| IBIS file generated by GenIBIS323.exe Version 3.23
|   TDA2Ex_23mm_abc
[IBIS ver]   5.0
[File name]   TDA2Ex_23mm_abc.ibs
[File Rev]   1.0.0
[Date]   Mon Apr 21, 2014, 15:13:32
[Source]   Data created at Texas Instruments
[Notes]   TDA2Ex_23mm 23mm IBIS Model Revision History
   Version 1.0.0, April 21, 2014
   - Initial Release
   Note 1) Checked by IBISCHK5.
   Note 2) Interfaces Included in this TDA2Ex_23mm 23x23 IBIS Model
   - EMIF1
   - GPIO6
   - GPMC
   - CSI
   - VIP2
   - DSS
   - HDMI1
   - RGMII
   - USB1,2
   - XREFCLK
   - McASP1,2,3,4,5
   - MMC1,3
   - SPI1,2
   - DCAN
   - UART1,2
   - SATA1
   - I2C1,2
   - MLB
   - PCIE
[Disclaimer] Please be aware that in the absence of a written agreement,
   Texas Instruments (TI) assumes no liability for: 1) the
   accuracy of the IBIS models provided to your company, 2) the
   proper functioning of these IBIS models in your design or for
   any resulting applications, or, 3) infringement of patents,
   copyrights, or intellectual property rights resulting from
   your use of these IBIS models. TI provides IBIS models as a
   service to our customers and therefore reserves the right to
   limit distribution of the IBIS models.
[Copyright]   Property of Texas Instruments Incorporated. Unauthorised
   reproduction and/or distribution is strictly prohibited. This
   product is protected under copyright law and trade secret law
   as an unpublished work. Created 2013,(C) Copyright 2013,
   Texas Instruments Incorporated., All Rights Reserved. These
   commodities are under the U.S. Government distribution license
   control.As such,they are not to be re-exported without the
   prior approval of the U.S. Department of Commerce.
|   Component TDA2Ex_23mm_abc
[Component]   TDA2Ex_23mm_abc
[Manufacturer]   Texas Instruments.
| Source IO level model revisions
|Model   Revision   Date
|ILVDS18HY_SSCEH   1.0   Apr 04, 2013
|BMLBLVDS18_SSCEH   1.0   Jun 13, 2013
|BC1833DV40DCPBFBP1811_SSCEH   2.0   Sep 11, 2013
|DDR_SEIOPB_H   2.4   14 Aug 2013
|GANGARX   1   Sep 04, 2012
|SDIO1833PB_H   1.0   Sep 21, 2011
|IQ1833DVTCKPBFBP18LL_SSCEV   2.0   Sep 11, 2013
|USB3_PCIEGEN1_PCIEGEN2_TX   1.0   Nov 07, 2012
|ACSPCIE_RX   0.5   May 16, 2012
|BI2C1833DVFZP18_SSCEV   2.0   Sep 11, 2013
|IHHV1833DVHYP1811_SSCEV   1.0   Dec 24, 2012
|DDR_SEIOPB_V   2.4   14 Aug 2013
|CAMERARX_CORE   0.9   March 31, 2014
|CAMERARX_ADDON   0.9   March 31, 2014
|DDR_DIFFIOPB_H   2.4   14 Aug 2013
|HDMITXPHY   0.8   Jul 12, 2011
|DDR_DIFFIOPB_V   2.4   14 Aug 2013
|BC1833DV40DCPBFBP1811_SSCEV   2.0   Sep 11, 2013
|USB2PHYCORE_HMAV10GS80   0.8   July 13, 2011
|SATATX   1.0   Nov 07, 2012
|BC1833DV40DCPBFBHHVRXP1811_SSCEV   2.0   Sep 11, 2013
[Package]
|   typ   min   max
R_pkg   0.537189936507937   9.1626E-02   1.1184E+00
L_pkg   7.79954444444445E-009 1.2113E-09   1.5606E-08
C_pkg   9.51173941798942E-013 3.9552E-13   1.7031E-12
[Pin]   signal_name   model_name   R_pin   L_pin   C_pin
Y10   ATESTV   NC
AG3   CSI2_0_DY4   Selector_16  8.5173E-01 1.2984E-08 1.1334E-12
AG6   CSI2_1_DX1   Selector_9   6.1027E-01 9.6063E-09 8.2820E-13
AH6   CSI2_1_DY1   Selector_14  6.0787E-01 1.0137E-08 8.5060E-13
AH5   CSI2_1_DY0   Selector_16  6.4591E-01 1.0727E-08 9.0708E-13
AH4   CSI2_0_DX3   Selector_21  7.1057E-01 1.1842E-08 1.0230E-12
AH3   CSI2_0_DX4   Selector_21  8.5056E-01 1.3007E-08 1.0794E-12
AF2   CSI2_0_DX2   Selector_9   7.2567E-01 1.2082E-08 9.7410E-13
AD2   CSI2_0_DY0   Selector_16  7.2276E-01 1.1113E-08 9.4758E-13
AG7   CSI2_1_DY2   Selector_14  5.6878E-01 8.9623E-09 7.3155E-13
AF1   CSI2_0_DX1   Selector_9   7.4892E-01 1.2381E-08 9.6375E-13
AG4   CSI2_0_DY3   Selector_16  7.0753E-01 1.1110E-08 9.4869E-13
AE1   CSI2_0_DX0   Selector_21  7.1918E-01 1.1582E-08 9.6996E-13
AG5   CSI2_1_DX0   Selector_21  6.4796E-01 1.0183E-08 8.8897E-13
AH7   CSI2_1_DX2   Selector_9   5.6894E-01 9.4930E-09 7.7235E-13
AF3   CSI2_0_DY2   Selector_14  7.2319E-01 1.1690E-08 9.4052E-13
AE2   CSI2_0_DY1   Selector_14  7.5166E-01 1.1989E-08 1.0007E-12
G20   DCAN1_TX   Selector_10  2.5712E-01 3.5844E-09 6.2646E-13
G19   DCAN1_RX   Selector_10  2.7051E-01 3.7171E-09 6.0175E-13
AA25   DDR1_D30   Selector_24  6.7015E-01 1.0040E-08 1.2856E-12
AH22   DDR1_A5   Selector_22  6.4123E-01 8.7087E-09 1.0685E-12
Y27   DDR1_DQSN3   Selector_8   6.2328E-01 1.0018E-08 8.4443E-13
AA26   DDR1_D29   Selector_24  6.6144E-01 9.6929E-09 1.1535E-12
Y25   DDR1_ECC_D4   Selector_24  6.5082E-01 1.0452E-08 1.1528E-12
AF23   DDR1_D6   Selector_24  6.7068E-01 9.7861E-09 1.1203E-12
AC26   DDR1_DQM2   Selector_25  6.4018E-01 9.4502E-09 9.6451E-13
AA27   DDR1_DQM3   Selector_25  6.7731E-01 1.0580E-08 9.8696E-13
AD20   DDR1_A0   Selector_22  6.6508E-01 5.9840E-09 9.7941E-13
W20   DDR1_D17   Selector_24  5.1391E-01 7.7161E-09 1.0916E-12
Y23   DDR1_D26   Selector_24  5.9348E-01 8.0574E-09 9.9265E-13
V20   DDR1_D16   Selector_24  5.6668E-01 6.3037E-09 1.0295E-12
AE28   DDR1_DQSN1   Selector_8   6.6530E-01 1.1238E-08 8.9885E-13
W22   DDR1_ECC_D0   Selector_24  5.5547E-01 8.9184E-09 1.0222E-12
Y20   DDR1_D23   Selector_24  5.5760E-01 7.3138E-09 8.6201E-13
AF25   DDR1_D0   Selector_24  6.9115E-01 1.0412E-08 1.0268E-12
AD27   DDR1_DQS2   Selector_5   6.4885E-01 1.0584E-08 9.0579E-13
AB18   DDR1_BA2   Selector_22  6.4393E-01 4.4937E-09 8.6957E-13
AD18   DDR1_A15   Selector_22  6.3880E-01 6.7930E-09 1.1482E-12
AH25   DDR1_DQS0   Selector_5   6.4552E-01 1.0566E-08 8.8659E-13
AF28   DDR1_D11   Selector_24  7.2153E-01 1.1434E-08 1.1074E-12
AC18   DDR1_CASN   Selector_22  6.8362E-01 5.3999E-09 7.8258E-13
AC17   DDR1_ODT1   Selector_25  2.8412E-01 4.0326E-09 6.1771E-13
AH21   DDR1_WEN   Selector_22  6.4749E-01 8.6863E-09 1.0744E-12
AC27   DDR1_D20   Selector_24  6.8065E-01 1.0127E-08 1.2395E-12
AA24   DDR1_D27   Selector_24  6.0442E-01 9.2946E-09 1.2881E-12
AC19   DDR1_A1   Selector_22  6.5278E-01 5.4173E-09 8.8612E-13
AE24   DDR1_D5   Selector_24  6.7685E-01 9.3912E-09 1.0978E-12
AF21   DDR1_A4   Selector_22  6.7313E-01 7.9943E-09 1.0791E-12
AE21   DDR1_A7   Selector_22  6.3854E-01 7.2344E-09 8.9151E-13
V25   DDR1_ECC_D6   Selector_24  6.6781E-01 9.7509E-09 1.1377E-12
V28   DDR1_DQSN_ECC   Selector_8   6.4251E-01 1.0836E-08 8.3093E-13
AH23   DDR1_CSN0   Selector_22  6.3626E-01 8.9469E-09 1.1247E-12
AE26   DDR1_D12   Selector_24  6.9974E-01 1.0254E-08 1.1468E-12
W19   DDR1_ECC_D2   Selector_24  5.1772E-01 8.4884E-09 9.8842E-13
AF27   DDR1_D9   Selector_24  6.8917E-01 1.0748E-08 1.1844E-12
V23   DDR1_ECC_D1   Selector_24  6.0789E-01 8.3957E-09 9.6847E-13
Y28   DDR1_DQS3   Selector_5   6.2753E-01 1.0576E-08 8.3228E-13
AB16   DDR1_CSN1   Selector_25  1.4691E-01 2.1740E-09 5.2457E-13
AF20   DDR1_RASN   Selector_22  6.4542E-01 7.3957E-09 9.2859E-13
AG24   DDR1_CK   Selector_23  6.1124E-01 9.4171E-09 8.8135E-13
AD28   DDR1_DQSN2   Selector_8   6.4587E-01 1.0864E-08 8.9563E-13
V24   DDR1_ECC_D5   Selector_24  6.1242E-01 9.0629E-09 1.1125E-12
AD23   DDR1_DQM0   Selector_25  7.0242E-01 7.8396E-09 8.4493E-13
AC21   DDR1_A12   Selector_22  6.3530E-01 5.5287E-09 7.8791E-13
Y18   DDR1_VREF0   NC
AF22   DDR1_A8   Selector_22  6.4839E-01 7.7909E-09 1.0176E-12
AF17   DDR1_BA0   Selector_22  5.6388E-01 6.8889E-09 1.2089E-12
AB27   DDR1_D22   Selector_24  6.8054E-01 9.9186E-09 1.1957E-12
AD25   DDR1_D15   Selector_24  6.6992E-01 1.0422E-08 9.8777E-13
W23   DDR1_ECC_D3   Selector_24  6.1842E-01 9.9342E-09 1.1360E-12
AB28   DDR1_D18   Selector_24  7.0422E-01 1.0354E-08 1.1122E-12
AF26   DDR1_D1   Selector_24  6.9734E-01 1.0561E-08 1.1454E-12
Y26   DDR1_ECC_D7   Selector_24  6.4468E-01 1.0660E-08 1.1202E-12
AG22   DDR1_CKE   Selector_22  6.3999E-01 8.4390E-09 1.1577E-12
AE27   DDR1_DQS1   Selector_5   6.6880E-01 1.1014E-08 9.4235E-13
AD21   DDR1_A10   Selector_22  6.4149E-01 6.3355E-09 1.0112E-12
AG21   DDR1_RST   Selector_22  6.3434E-01 8.3979E-09 1.0138E-12
AG27   DDR1_D10   Selector_24  7.2020E-01 1.1407E-08 1.1486E-12
Y22   DDR1_D25   Selector_24  5.9804E-01 7.9738E-09 1.0895E-12
AE20   DDR1_ODT0   Selector_22  6.3872E-01 6.9316E-09 9.3687E-13
AG25   DDR1_DQSN0   Selector_8   6.4270E-01 1.0163E-08 9.1809E-13
AC24   DDR1_D14   Selector_24  6.5703E-01 9.2646E-09 1.1109E-12
AD22   DDR1_A11   Selector_22  6.7006E-01 6.8570E-09 8.1281E-13
V26   DDR1_DQM_ECC   Selector_25  6.4924E-01 1.0064E-08 9.3962E-13
AE17   DDR1_A14   Selector_22  6.2767E-01 6.2691E-09 8.5084E-13
AC20   DDR1_A2   Selector_22  6.3389E-01 5.7286E-09 9.3968E-13
AE22   DDR1_A9   Selector_22  6.4601E-01 6.9701E-09 9.6295E-13
AC25   DDR1_D13   Selector_24  7.0800E-01 9.9894E-09 1.1340E-12
AH26   DDR1_D3   Selector_24  7.0980E-01 1.1203E-08 1.1710E-12
AG23   DDR1_A6   Selector_22  6.4214E-01 8.8818E-09 1.0053E-12
AF24   DDR1_D4   Selector_24  7.0560E-01 1.0213E-08 1.2143E-12
AA28   DDR1_D31   Selector_24  6.6814E-01 1.0601E-08 1.1364E-12
AB19   DDR1_A3   Selector_22  6.8082E-01 4.7400E-09 9.7992E-13
Y24   DDR1_D28   Selector_24  6.3912E-01 9.2036E-09 1.2543E-12
V27   DDR1_DQS_ECC   Selector_5   6.4069E-01 1.0727E-08 8.3511E-13
AA23   DDR1_D24   Selector_24  6.3577E-01 9.4352E-09 1.1967E-12
AH24   DDR1_NCK   Selector_19  6.0644E-01 9.5797E-09 8.5394E-13
AB23   DDR1_DQM1   Selector_25  6.8934E-01 8.7385E-09 9.9142E-13
Y19   DDR1_D21   Selector_24  5.0560E-01 8.1840E-09 1.0160E-12
AG26   DDR1_D2   Selector_24  7.1707E-01 1.1027E-08 1.1977E-12
AF18   DDR1_A13   Selector_22  6.3499E-01 6.7548E-09 1.1981E-12
AC23   DDR1_D8   Selector_24  6.8672E-01 9.1685E-09 1.0928E-12
AE18   DDR1_BA1   Selector_22  6.3547E-01 6.1764E-09 1.0753E-12
AC28   DDR1_D19   Selector_24  6.9091E-01 1.0396E-08 1.2165E-12
AE23   DDR1_D7   Selector_24  6.8260E-01 8.9564E-09 1.0358E-12
G21   EMU0   Selector_10  2.9273E-01 4.0267E-09 6.8795E-13
D24   EMU1   Selector_10  9.6844E-01 1.2920E-08 1.4586E-12
F21   GPIO6_16   Selector_10  4.5597E-01 6.7483E-09 9.4581E-13
E21   GPIO6_14   Selector_10  4.3851E-01 6.0672E-09 9.1248E-13
AC5   GPIO6_10   Selector_4   5.8226E-01 8.0653E-09 1.0821E-12
AB4   GPIO6_11   Selector_4   5.3537E-01 7.3814E-09 1.0901E-12
F20   GPIO6_15   Selector_10  3.5541E-01 5.0224E-09 8.3644E-13
K2   GPMC_AD9   Selector_4   4.5105E-01 6.7623E-09 8.5620E-13
K6   GPMC_A22   Selector_4   2.5324E-01 3.3932E-09 5.4317E-13
J4   GPMC_A24   Selector_4   3.5558E-01 5.2045E-09 7.2229E-13
J3   GPMC_AD13   Selector_4   4.1235E-01 6.0344E-09 8.6798E-13
R6   GPMC_A0   Selector_4   2.7951E-01 3.8456E-09 6.7724E-13
P3   GPMC_A17   Selector_4   4.6557E-01 6.7082E-09 9.5834E-13
L1   GPMC_AD8   Selector_4   5.4155E-01 8.1549E-09 9.7489E-13
L5   GPMC_AD2   Selector_4   3.0148E-01 4.2442E-09 6.6311E-13
P6   GPMC_A4   Selector_4   2.5737E-01 3.4048E-09 6.7625E-13
P5   GPMC_A7   Selector_4   3.1377E-01 4.2556E-09 7.4241E-13
M7   GPMC_A20   Selector_4   2.3964E-01 3.9225E-09 6.3833E-13
P1   GPMC_CS3   Selector_4   5.7518E-01 8.5305E-09 1.0491E-12
R3   GPMC_A13   Selector_4   4.4827E-01 6.4852E-09 9.8152E-13
L4   GPMC_AD5   Selector_4   3.2349E-01 4.6692E-09 7.1767E-13
H5   GPMC_A27   Selector_4   3.4218E-01 4.8457E-09 7.1178E-13
T9   GPMC_A1   Selector_4   3.4531E-01 4.5998E-09 8.3332E-13
P4   GPMC_A12   Selector_4   3.9853E-01 5.4982E-09 8.4479E-13
M1   GPMC_AD3   Selector_4   5.3504E-01 7.9023E-09 8.0504E-13
J1   GPMC_AD10   Selector_4   5.6454E-01 8.4119E-09 9.4862E-13
R2   GPMC_A18   Selector_4   5.1527E-01 7.5891E-09 1.0050E-12
M2   GPMC_AD1   Selector_4   4.5542E-01 6.8146E-09 7.5204E-13
H2   GPMC_AD14   Selector_4   5.2793E-01 7.7543E-09 1.0096E-12
N6   GPMC_BEN0   Selector_4   2.2301E-01 3.0227E-09 6.2122E-13
M6   GPMC_AD0   Selector_4   2.5765E-01 3.5537E-09 6.3279E-13
J6   GPMC_A25   Selector_4   2.8546E-01 3.9342E-09 6.7657E-13
R4   GPMC_A9   Selector_4   3.9804E-01 5.5259E-09 7.7746E-13
N9   GPMC_A10   Selector_4   9.1626E-02 1.2113E-09 3.9552E-13
L6   GPMC_AD4   Selector_4   2.4365E-01 3.4502E-09 6.1430E-13
R5   GPMC_A6   Selector_4   3.7488E-01 5.0526E-09 7.8998E-13
M4   GPMC_BEN1   Selector_4   3.6085E-01 5.2185E-09 7.5404E-13
J5   GPMC_A21   Selector_4   2.9678E-01 4.1954E-09 5.8522E-13
P7   GPMC_CLK   Selector_4   2.0670E-01 2.7146E-09 5.0835E-13
J2   GPMC_AD11   Selector_4   4.7926E-01 7.1453E-09 9.9013E-13
T1   GPMC_CS0   Selector_4   6.1706E-01 9.1439E-09 1.0538E-12
H1   GPMC_AD12   Selector_4   5.9408E-01 8.8427E-09 1.0004E-12
T6   GPMC_A2   Selector_4   3.8093E-01 5.2046E-09 8.3363E-13
T2   GPMC_A14   Selector_4   5.4930E-01 8.0763E-09 1.0296E-12
H6   GPMC_CS1   Selector_4   3.0615E-01 4.1656E-09 7.0997E-13
H3   GPMC_AD15   Selector_4   4.6620E-01 6.7682E-09 7.9782E-13
U2   GPMC_A15   Selector_4   5.8453E-01 8.6503E-09 1.1275E-12
N1   GPMC_ADVN_ALE   Selector_4   5.3053E-01 7.9787E-09 8.4211E-13
N2   GPMC_WAIT0   Selector_4   5.0546E-01 7.5397E-09 9.1702E-13
N7   GPMC_A8   Selector_4   2.1276E-01 2.5701E-09 5.6699E-13
K7   GPMC_A19   Selector_4   1.8753E-01 2.5304E-09 4.6060E-13
J7   GPMC_A23   Selector_4   2.0556E-01 2.6865E-09 5.5900E-13
T7   GPMC_A3   Selector_4   3.5841E-01 5.0548E-09 9.1406E-13
M3   GPMC_WEN   Selector_4   4.1189E-01 6.0280E-09 7.7365E-13
U1   GPMC_A16   Selector_4   6.5653E-01 9.6078E-09 1.1885E-12
R9   GPMC_A5   Selector_4   2.5272E-01 3.4335E-09 7.7845E-13
P9   GPMC_A11   Selector_4   1.2100E-01 1.5460E-09 5.1701E-13
L3   GPMC_AD6   Selector_4   4.1570E-01 6.0691E-09 8.6239E-13
L2   GPMC_AD7   Selector_4   4.4867E-01 6.6660E-09 9.4487E-13
H4   GPMC_A26   Selector_4   4.0521E-01 5.7228E-09 7.8712E-13
M5   GPMC_OEN_REN   Selector_4   2.8852E-01 4.0933E-09 6.5541E-13
P2   GPMC_CS2   Selector_4   4.9624E-01 7.3225E-09 1.0296E-12
AH16   HDMI1_CLOCKY   Model_576   5.1119E-01 7.7388E-09 6.9914E-13
AH17   HDMI1_DATA0Y   Model_576   5.2733E-01 7.8951E-09 7.1265E-13
AH19   HDMI1_DATA2Y   Model_576   5.7556E-01 8.5919E-09 7.4180E-13
AH18   HDMI1_DATA1Y   Model_576   5.4131E-01 8.2130E-09 7.3367E-13
AG16   HDMI1_CLOCKX   Model_575   5.1455E-01 7.3206E-09 6.7496E-13
AG18   HDMI1_DATA1X   Model_575   5.3868E-01 7.7198E-09 7.3337E-13
AG19   HDMI1_DATA2X   Model_575   5.7564E-01 8.0628E-09 7.4733E-13
AG17   HDMI1_DATA0X   Model_575   5.3126E-01 7.5769E-09 7.1991E-13
F17   I2C2_SCL   Selector_3   2.8851E-01 3.9932E-09 7.0332E-13
C21   I2C1_SDA   Selector_3   4.6380E-01 6.4148E-09 9.2034E-13
C20   I2C1_SCL   Selector_3   4.4242E-01 6.1907E-09 9.3364E-13
C25   I2C2_SDA   Selector_3   8.6423E-01 1.1725E-08 1.4162E-12
AG15   LJCB_CLKP   Model_228   5.3615E-01 7.9977E-09 7.4012E-13
AH15   LJCB_CLKN   Model_228   5.3802E-01 8.3516E-09 7.5042E-13
E12   MCASP1_AXR4   Selector_10  3.7755E-01 5.3040E-09 7.4370E-13
B14   MCASP1_ACLKR   Selector_10  4.8051E-01 7.1622E-09 8.6398E-13
G13   MCASP1_AXR2   Selector_10  2.1814E-01 2.9073E-09 6.0717E-13
A11   MCASP1_AXR9   Selector_10  6.3097E-01 9.2337E-09 1.0375E-12
G12   MCASP1_AXR0   Selector_10  1.7167E-01 3.1362E-09 5.6933E-13
D14   MCASP1_FSX   Selector_10  3.5358E-01 5.1483E-09 7.3643E-13
G14   MCASP1_AXR14   Selector_10  2.3781E-01 3.1899E-09 6.4652E-13
A13   MCASP1_AXR13   Selector_10  5.6674E-01 8.4060E-09 9.1156E-13
F13   MCASP1_AXR5   Selector_10  2.9281E-01 3.9652E-09 6.4956E-13
D12   MCASP1_AXR7   Selector_10  4.2870E-01 6.0720E-09 8.2704E-13
F12   MCASP1_AXR1   Selector_10  2.8745E-01 4.0444E-09 6.8891E-13
J14   MCASP1_FSR   Selector_10  1.6618E-01 2.5143E-09 6.3040E-13
B13   MCASP1_AXR10   Selector_10  5.2540E-01 7.5316E-09 9.3833E-13
C12   MCASP1_AXR6   Selector_10  4.6453E-01 6.6439E-09 8.8978E-13
E14   MCASP1_AXR12   Selector_10  3.0651E-01 4.2828E-09 7.0185E-13
B12   MCASP1_AXR8   Selector_10  5.2273E-01 7.6049E-09 9.9581E-13
F14   MCASP1_AXR15   Selector_10  2.9026E-01 3.9213E-09 6.7821E-13
J11   MCASP1_AXR3   Selector_10  2.2012E-01 4.1883E-09 7.0892E-13
A12   MCASP1_AXR11   Selector_10  5.8140E-01 8.5233E-09 9.3184E-13
C14   MCASP1_ACLKX   Selector_10  4.3412E-01 6.2886E-09 8.2460E-13
A16   MCASP2_AXR3   Selector_10  5.3849E-01 7.8845E-09 9.5182E-13
A19   MCASP2_ACLKX   Selector_10  6.5845E-01 9.3007E-09 1.0728E-12
E15   MCASP2_ACLKR   Selector_10  3.5749E-01 4.8677E-09 7.9261E-13
D15   MCASP2_AXR4   Selector_10  3.6671E-01 5.2518E-09 7.7018E-13
B17   MCASP2_AXR6   Selector_10  4.9306E-01 7.1674E-09 8.8919E-13
C15   MCASP2_AXR2   Selector_10  4.3354E-01 6.1885E-09 8.5537E-13
B15   MCASP2_AXR0   Selector_10  5.1629E-01 7.5166E-09 9.4345E-13
A18   MCASP2_FSX   Selector_10  5.9676E-01 8.6733E-09 1.1341E-12
A17   MCASP2_AXR7   Selector_10  5.6934E-01 8.3254E-09 9.4976E-13
B16   MCASP2_AXR5   Selector_10  5.1306E-01 7.4029E-09 9.4316E-13
A20   MCASP2_FSR   Selector_10  6.6258E-01 9.5504E-09 1.0850E-12
A15   MCASP2_AXR1   Selector_10  5.4609E-01 8.0020E-09 9.0744E-13
C17   MCASP3_AXR1   Selector_10  4.7040E-01 6.7643E-09 9.0007E-13
F15   MCASP3_FSX   Selector_10  2.6137E-01 3.7823E-09 7.3331E-13
B19   MCASP3_AXR0   Selector_10  5.6533E-01 8.0738E-09 9.5581E-13
B18   MCASP3_ACLKX   Selector_10  5.4440E-01 7.7902E-09 1.0570E-12
A21   MCASP4_FSX   Selector_10  6.9745E-01 1.0005E-08 1.1140E-12
D17   MCASP4_AXR1   Selector_10  3.8892E-01 5.2944E-09 7.8991E-13
C18   MCASP4_ACLKX   Selector_10  4.5617E-01 6.4207E-09 8.9604E-13
G16   MCASP4_AXR0   Selector_10  2.2931E-01 2.9043E-09 6.0837E-13
AB3   MCASP5_AXR0   Selector_4   6.5892E-01 9.0230E-09 1.1592E-12
AB9   MCASP5_FSX   Selector_4   2.4358E-01 4.2860E-09 8.6924E-13
AA3   MCASP5_ACLKX   Selector_4   5.5637E-01 7.6919E-09 1.1521E-12
AA4   MCASP5_AXR1   Selector_4   5.2316E-01 6.9325E-09 1.1006E-12
U4   MDIO_D   Selector_4   4.6376E-01 6.5098E-09 8.3538E-13
V1   MDIO_MCLK   Selector_4   6.0512E-01 8.7822E-09 8.5397E-13
AA1   MLBP_DAT_P   Selector_26  6.6785E-01 9.6958E-09 1.1029E-12
AB2   MLBP_CLK_N   Selector_17  7.2417E-01 1.0366E-08 1.0549E-12
AC2   MLBP_SIG_N   Selector_26  7.6446E-01 1.1061E-08 1.2378E-12
AA2   MLBP_DAT_N   Selector_26  6.6965E-01 9.5322E-09 1.1817E-12
AB1   MLBP_CLK_P   Selector_17  7.2333E-01 1.0563E-08 1.0127E-12
AC1   MLBP_SIG_P   Selector_26  7.6336E-01 1.1204E-08 1.2256E-12
W6   MMC1_CLK   Selector_7   3.0071E-01 4.2321E-09 6.2185E-13
Y3   MMC1_DAT3   Selector_7   5.0400E-01 7.3040E-09 9.1373E-13
AA6   MMC1_DAT0   Selector_7   5.4348E-01 7.6188E-09 1.0720E-12
Y4   MMC1_DAT1   Selector_7   4.5048E-01 6.4446E-09 9.5940E-13
W7   MMC1_SDCD   Selector_4   2.7015E-01 3.7095E-09 7.3413E-13
Y9   MMC1_SDWP   Selector_4   1.8078E-01 3.0393E-09 7.1707E-13
Y5   MMC1_BIAS   NC
AA5   MMC1_DAT2   Selector_7   6.0054E-01 8.1162E-09 1.1515E-12
Y6   MMC1_CMD   Selector_7   4.2844E-01 6.1549E-09 9.5233E-13
AC4   MMC3_CMD   Selector_4   5.6386E-01 7.8122E-09 1.1165E-12
AC7   MMC3_DAT0   Selector_4   4.7815E-01 9.1052E-09 1.5306E-12
AC9   MMC3_DAT2   Selector_4   3.0708E-01 5.7298E-09 9.1099E-13
AB8   MMC3_DAT6   Selector_4   2.7158E-01 4.8212E-09 8.4352E-13
AC3   MMC3_DAT3   Selector_4   6.1633E-01 8.6919E-09 1.1150E-12
AD4   MMC3_CLK   Selector_4   6.7013E-01 9.3348E-09 9.5526E-13
AD6   MMC3_DAT5   Selector_4   5.8554E-01 1.1841E-08 1.7031E-12
AC8   MMC3_DAT4   Selector_4   5.0066E-01 9.4255E-09 1.4698E-12
AC6   MMC3_DAT1   Selector_4   5.1802E-01 9.8492E-09 1.6746E-12
AB5   MMC3_DAT7   Selector_4   4.8522E-01 6.6868E-09 7.8256E-13
D21   NMIN   Selector_18  7.2536E-01 1.1044E-08 1.1466E-12
Y11   ON_OFF   Selector_11  1.6181E-01 2.8073E-09 5.4896E-13
AH14   PCIE_TXP0   Selector_6   4.9113E-01 7.9046E-09 7.1384E-13
AG13   PCIE_RXN0   Model_177   4.8705E-01 7.4410E-09 6.7416E-13
AH13   PCIE_RXP0   Model_177   4.8890E-01 7.9079E-09 6.8859E-13
AG14   PCIE_TXN0   Selector_2   4.8911E-01 7.4597E-09 7.0696E-13
F22   PORZ   Selector_12  4.9016E-01 7.1155E-09 8.4616E-13
E23   RESETN   Selector_18  5.3146E-01 8.2117E-09 7.3315E-13
V5   RGMII0_RXCTL   Selector_4   5.0418E-01 6.3130E-09 9.1001E-13
V4   RGMII0_RXD3   Selector_4   4.9545E-01 6.4890E-09 9.8511E-13
U5   RGMII0_RXC   Selector_4   4.8523E-01 5.9733E-09 1.0396E-12
V6   RGMII0_TXD1   Selector_4   3.9397E-01 5.4071E-09 9.4121E-13
W9   RGMII0_TXC   Selector_4   3.3651E-01 4.8996E-09 9.5485E-13
V3   RGMII0_RXD2   Selector_4   5.1126E-01 7.1551E-09 1.1082E-12
Y2   RGMII0_RXD1   Selector_4   6.0853E-01 8.6814E-09 1.2153E-12
U7   RGMII0_TXD2   Selector_4   2.9925E-01 3.8763E-09 8.8166E-13
V9   RGMII0_TXCTL   Selector_4   2.3299E-01 3.6162E-09 9.4166E-13
U6   RGMII0_TXD0   Selector_4   3.4453E-01 4.4298E-09 8.0265E-13
V7   RGMII0_TXD3   Selector_4   3.0414E-01 4.4394E-09 9.0935E-13
W2   RGMII0_RXD0   Selector_4   5.8414E-01 8.2072E-09 1.0059E-12
U3   RMII_MHZ_50_CLK   Selector_4   4.8927E-01 6.8487E-09 8.6355E-13
F23   RSTOUTN   Selector_13  4.6249E-01 7.2165E-09 7.6827E-13
AB17   RTC_PORZ   Selector_12  1.7244E-01 3.1812E-09 5.8735E-13
AE14   RTC_OSC_XI_CLKIN32   NC
AD14   RTC_OSC_XO   NC
AF14   RTC_ISO   Selector_12  4.2304E-01 5.9110E-09 7.7551E-13
E18   RTCK   Selector_13  7.8651E-01 1.2545E-08 1.4198E-12
AH10   SATA1_TXP0   Model_761   5.7455E-01 8.8354E-09 7.8211E-13
AG10   SATA1_TXN0   Model_761   5.7231E-01 8.4567E-09 7.6011E-13
AG9   SATA1_RXP0   Model_177   5.9393E-01 8.7588E-09 7.7850E-13
AH9   SATA1_RXN0   Model_177   5.9610E-01 9.1380E-09 7.8332E-13
B20   SPI1_CS3   Selector_10  4.8253E-01 7.0440E-09 9.8815E-13
B21   SPI1_CS2   Selector_10  7.1554E-01 9.4534E-09 1.3392E-12
A22   SPI1_CS1   Selector_10  7.8430E-01 1.0569E-08 1.3435E-12
A24   SPI1_CS0   Selector_10  9.8724E-01 1.3446E-08 1.2779E-12
A25   SPI1_SCLK   Selector_10  9.7089E-01 1.3378E-08 1.5964E-12
F16   SPI1_D1   Selector_10  3.0413E-01 4.3266E-09 6.5561E-13
B25   SPI1_D0   Selector_10  9.4783E-01 1.2659E-08 1.5659E-12
B24   SPI2_CS0   Selector_10  8.3497E-01 1.1899E-08 1.2403E-12
A26   SPI2_SCLK   Selector_10  1.0798E+00 1.5351E-08 1.5499E-12
G17   SPI2_D0   Selector_10  3.2480E-01 5.7521E-09 7.4295E-13
B22   SPI2_D1   Selector_10  6.6582E-01 9.7971E-09 1.0965E-12
E20   TCLK   Selector_15  5.2788E-01 7.1160E-09 8.7671E-13
D23   TDI   Selector_18  7.6631E-01 1.0647E-08 1.2045E-12
F19   TDO   Selector_13  6.1661E-01 1.0487E-08 1.1261E-12
F18   TMS   Selector_18  5.1753E-01 9.1264E-09 1.0325E-12
D20   TRSTN   Selector_18  7.6834E-01 1.1481E-08 1.1840E-12
C27   UART1_RTSN   Selector_10  8.0845E-01 1.3380E-08 1.3207E-12
C26   UART1_TXD   Selector_10  7.6368E-01 1.2561E-08 1.1873E-12
B27   UART1_RXD   Selector_10  8.3517E-01 1.3765E-08 1.2671E-12
E25   UART1_CTSN   Selector_10  6.4386E-01 1.0595E-08 1.0162E-12
D27   UART2_CTSN   Selector_10  7.5421E-01 1.2875E-08 1.0257E-12
C28   UART2_RTSN   Selector_10  8.7534E-01 1.4335E-08 1.4113E-12
D28   UART2_RXD   Selector_10  8.0475E-01 1.3445E-08 1.1920E-12
D26   UART2_TXD   Selector_10  7.2598E-01 1.2154E-08 1.2260E-12
V2   UART3_RXD   Selector_4   5.5046E-01 7.7610E-09 1.1171E-12
Y1   UART3_TXD   Selector_4   6.8457E-01 9.7714E-09 1.1857E-12
AC11   USB_TXN0   Selector_2   2.2294E-01 3.4058E-09 5.1726E-13
AF12   USB_RXN0   Model_177   4.0618E-01 6.2457E-09 6.1259E-13
AE12   USB_RXP0   Model_177   4.0350E-01 5.7509E-09 5.9805E-13
AD11   USB_TXP0   Selector_6   2.2477E-01 3.5787E-09 7.5073E-13
AB10   USB1_DRVVBUS   Selector_4   2.1393E-01 3.9628E-09 7.0827E-13
AD12   USB1_DP   Selector_20  3.2235E-01 5.0848E-09 6.3358E-13
AC12   USB1_DM   Selector_1   3.2040E-01 4.8693E-09 8.2475E-13
AC10   USB2_DRVVBUS   Selector_4   2.4048E-01 4.6878E-09 9.4598E-13
AF11   USB2_DM   Selector_1   3.8946E-01 6.2321E-09 5.9426E-13
AE11   USB2_DP   Selector_20  3.8657E-01 5.8729E-09 6.1806E-13
B5   VIN2A_D22   Selector_10  6.5334E-01 9.7358E-09 1.2697E-12
G6   VIN2A_VSYNC0   Selector_10  3.4152E-01 4.8728E-09 7.4139E-13
D5   VIN2A_D12   Selector_10  5.9498E-01 8.6494E-09 1.0373E-12
D2   VIN2A_D4   Selector_10  7.7295E-01 1.0944E-08 1.3108E-12
C4   VIN2A_D15   Selector_10  6.4211E-01 9.6502E-09 1.2301E-12
E4   VIN2A_D7   Selector_10  5.4410E-01 8.0421E-09 9.7268E-13
C5   VIN2A_D18   Selector_10  6.3043E-01 9.2777E-09 1.1141E-12
B4   VIN2A_D21   Selector_10  7.1886E-01 1.0722E-08 1.3749E-12
D6   VIN2A_D17   Selector_10  5.0796E-01 7.5327E-09 9.8829E-13
E2   VIN2A_D3   Selector_10  6.5148E-01 9.5942E-09 1.2265E-12
F6   VIN2A_D11   Selector_10  4.2375E-01 6.2040E-09 8.7025E-13
G2   VIN2A_DE0   Selector_10  5.6165E-01 8.3476E-09 9.9641E-13
G1   VIN2A_HSYNC0   Selector_10  6.0809E-01 9.0931E-09 1.0216E-12
A4   VIN2A_D23   Selector_10  7.6105E-01 1.1364E-08 1.2158E-12
F3   VIN2A_D1   Selector_10  5.4193E-01 7.9726E-09 1.1026E-12
F4   VIN2A_D5   Selector_10  5.5693E-01 7.9511E-09 1.0735E-12
E1   VIN2A_CLK0   Selector_10  6.7228E-01 1.0162E-08 8.5927E-13
B3   VIN2A_D20   Selector_10  7.6005E-01 1.1365E-08 1.3420E-12
A3   VIN2A_D19   Selector_10  7.8456E-01 1.1783E-08 1.3796E-12
C2   VIN2A_D13   Selector_10  7.4634E-01 1.1209E-08 1.3944E-12
C1   VIN2A_D6   Selector_10  8.0223E-01 1.1882E-08 1.2614E-12
F2   VIN2A_D0   Selector_10  6.2608E-01 9.2902E-09 9.2254E-13
C3   VIN2A_D14   Selector_10  7.1727E-01 1.0652E-08 1.2328E-12
B2   VIN2A_D16   Selector_10  8.1320E-01 1.2175E-08 1.3522E-12
E6   VIN2A_D9   Selector_10  4.6448E-01 6.6995E-09 9.2775E-13
D3   VIN2A_D10   Selector_10  6.7115E-01 9.9545E-09 1.0537E-12
D1   VIN2A_D2   Selector_10  7.6059E-01 1.1156E-08 1.1853E-12
H7   VIN2A_FLD0   Selector_10  2.6110E-01 3.4827E-09 6.2503E-13
F5   VIN2A_D8   Selector_10  4.9168E-01 7.0305E-09 9.5166E-13
A8   VOUT1_D19   Selector_10  6.2923E-01 9.5740E-09 1.0738E-12
F8   VOUT1_D6   Selector_10  4.9472E-01 6.9757E-09 9.2975E-13
B9   VOUT1_D22   Selector_10  6.0266E-01 8.6928E-09 1.0955E-12
E11   VOUT1_VSYNC   Selector_10  4.1396E-01 5.8761E-09 8.2178E-13
C7   VOUT1_D15   Selector_10  5.9817E-01 9.0204E-09 1.0720E-12
F10   VOUT1_D2   Selector_10  3.0980E-01 4.2410E-09 6.9951E-13
F9   VOUT1_D5   Selector_10  3.7659E-01 5.1141E-09 7.4936E-13
C9   VOUT1_D20   Selector_10  5.3224E-01 7.7930E-09 1.0411E-12
D9   VOUT1_D9   Selector_10  6.4803E-01 8.7422E-09 1.1010E-12
A5   VOUT1_D12   Selector_10  8.2004E-01 1.2125E-08 1.2766E-12
F11   VOUT1_D0   Selector_10  2.5456E-01 3.4428E-09 6.6543E-13
A9   VOUT1_D21   Selector_10  6.3518E-01 9.3167E-09 1.0770E-12
A10   VOUT1_D23   Selector_10  5.8797E-01 8.7403E-09 1.0476E-12
C11   VOUT1_HSYNC   Selector_10  4.6779E-01 6.8214E-09 8.5828E-13
C8   VOUT1_D14   Selector_10  5.6673E-01 8.4027E-09 1.0772E-12
E7   VOUT1_D7   Selector_10  5.2295E-01 7.6736E-09 1.0169E-12
D8   VOUT1_D11   Selector_10  4.8819E-01 7.3058E-09 9.3082E-13
B8   VOUT1_D17   Selector_10  5.8039E-01 8.7920E-09 1.1608E-12
G11   VOUT1_D3   Selector_10  1.1612E-01 2.3504E-09 5.6954E-13
B7   VOUT1_D16   Selector_10  6.6100E-01 9.9435E-09 1.1220E-12
B11   VOUT1_FLD   Selector_10  5.1498E-01 7.6825E-09 9.4578E-13
B10   VOUT1_DE   Selector_10  5.6204E-01 8.2766E-09 9.5154E-13
D7   VOUT1_D10   Selector_10  5.8104E-01 8.4982E-09 1.0462E-12
A7   VOUT1_D18   Selector_10  7.0122E-01 1.0648E-08 1.1552E-12
D11   VOUT1_CLK   Selector_10  4.0193E-01 5.8263E-09 7.1584E-13
E8   VOUT1_D8   Selector_10  4.5892E-01 6.6144E-09 8.9060E-13
E9   VOUT1_D4   Selector_10  3.8282E-01 5.5621E-09 7.6089E-13
C6   VOUT1_D13   Selector_10  6.4327E-01 9.6650E-09 1.2094E-12
G10   VOUT1_D1   Selector_10  3.1695E-01 4.1725E-09 6.7884E-13
AD17   WAKEUP0   Selector_12  4.4712E-01 6.6884E-09 8.8622E-13
AC16   WAKEUP3   Selector_12  2.8200E-01 3.7672E-09 7.2803E-13
AE15   XI_OSC0   NC
AC15   XI_OSC1   NC
AD15   XO_OSC0   NC
AC13   XO_OSC1   NC
C23   XREF_CLK3   Selector_10  7.3470E-01 1.0531E-08 1.0284E-12
D18   XREF_CLK0   Selector_10  4.9128E-01 8.4217E-09 1.0131E-12
B26   XREF_CLK2   Selector_10  1.1184E+00 1.5606E-08 1.3887E-12
E17   XREF_CLK1   Selector_10  4.3541E-01 7.9076E-09 9.3080E-13
[Diff Pin] inv_pin vdiff tdelay_typ tdelay_min tdelay_max
|Differential signal data for cell CAMERARX_CORE
|CSI2_0_DX1   CSI2_0_DY1
AF1   AE2   200m   NA
|CSI2_1_DX2   CSI2_1_DY2
AH7   AG7   200m   NA
|CSI2_0_DX2   CSI2_0_DY2
AF2   AF3   200m   NA
|CSI2_1_DX1   CSI2_1_DY1
AG6   AH6   200m   NA
|Differential signal data for cell ILVDS18HY_SSCEH
|MLBP_CLK_P   MLBP_CLK_N
AB1   AB2   200m   NA
|Differential signal data for cell BMLBLVDS18_SSCEH
|MLBP_SIG_P   MLBP_SIG_N
AC1   AC2   200m   NA
|MLBP_DAT_P   MLBP_DAT_N
AA1   AA2   200m   NA
|Differential signal data for cell CAMERARX_ADDON
|CSI2_1_DX0   CSI2_1_DY0
AG5   AH5   200m   NA
|CSI2_0_DX4   CSI2_0_DY4
AH3   AG3   200m   NA
|CSI2_0_DX3   CSI2_0_DY3
AH4   AG4   200m   NA
|CSI2_0_DX0   CSI2_0_DY0
AE1   AD2   200m   NA
|Differential signal data for cell GANGARX
|PCIE_RXP0   PCIE_RXN0
AH13   AG13   100mV  NA
|SATA1_RXP0   SATA1_RXN0
AG9   AH9   100mV  NA
|USB_RXP0   USB_RXN0
AE12   AF12   100mV  NA
|Differential signal data for cell DDR_DIFFIOPB_H
|DDR1_DQS0   DDR1_DQSN0
AH25   AG25   200m   0
|DDR1_DQS3   DDR1_DQSN3
Y28   Y27   200m   0
|DDR1_DQS_ECC   DDR1_DQSN_ECC
V27   V28   200m   0
|DDR1_DQS1   DDR1_DQSN1
AE27   AE28   200m   0
|DDR1_DQS2   DDR1_DQSN2
AD27   AD28   200m   0
|Differential signal data for cell USB3_PCIEGEN1_PCIEGEN2_TX
|USB_TXP0   USB_TXN0
AD11   AC11   200m   0
|PCIE_TXP0   PCIE_TXN0
AH14   AG14   200m   0
|Differential signal data for cell HDMITXPHY
|HDMI1_DATA0X   HDMI1_DATA0Y
AG17   AH17   0.0V   0.0s
|HDMI1_DATA2X   HDMI1_DATA2Y
AG19   AH19   0.0V   0.0s
|HDMI1_CLOCKX   HDMI1_CLOCKY
AG16   AH16   0.0V   0.0s
|HDMI1_DATA1X   HDMI1_DATA1Y
AG18   AH18   0.0V   0.0s
|Differential signal data for cell DDR_DIFFIOPB_V
|DDR1_CK   DDR1_NCK
AG24   AH24   200m   0
|Differential signal data for cell ACSPCIE_RX
|LJCB_CLKP   LJCB_CLKN
AG15   AH15   150m   NA   NA   NA
|Differential signal data for cell USB2PHYCORE_HMAV10GS80
|USB1_DP   USB1_DM
AD12   AC12   200mV 0ns 0ns 0ns
|USB2_DP   USB2_DM
AE11   AF11   200mV 0ns 0ns 0ns
|Differential signal data for cell SATATX
|SATA1_TXP0   SATA1_TXN0
AH10   AG10   200m   0
|   Usage I/O#X###USB2PHYCORE_HMAV10GS80.DM
|   Base model USB2PHYCORE_HMAV10GS80
[Model Selector] Selector_1
Model_739 3-STATE,3.3000V,fsdm_tx
Model_741 3-STATE,3.3000V,lsdm_50pf_tx
Model_743 3-STATE,3.3000V,lsdm_200pf_tx
Model_745 3-STATE,3.3000V,lsdm_400pf_tx
Model_747 3-STATE,3.3000V,lsdm_600pf_tx
Model_748 INPUT,3.3V,fsrx
Model_750 3-STATE,0.8000V,hsdm_tx
Model_751 INPUT,3.3V,hsrx
|   Usage OUTPUT#X###USB3_PCIEGEN1_PCIEGEN2_TX.TXN
|   Base model USB3_PCIEGEN1_PCIEGEN2_TX
[Model Selector] Selector_2
Model_190 3-STATE,1.1V,USB3_TX_FS_NO_DEEMPHASIS
Model_191 3-STATE,1.1V,USB3_TX_FS_3p5_DEEMPHASIS
Model_192 3-STATE,1.1V,USB3_TX_HS_NO_DEEMPHASIS
Model_193 3-STATE,1.1V,PCIEGEN1_TX_FS_NO_DEEMPHASIS_1p2v
Model_194 3-STATE,1.1V,PCIEGEN1_TX_FS_NO_DEEMPHASIS_0p8v
Model_195 3-STATE,1.1V,PCIEGEN1_TX_FS_NO_DEEMPHASIS_0p6v
Model_196 3-STATE,1.1V,PCIEGEN1_TX_FS_NO_DEEMPHASIS_0p4v
Model_197 3-STATE,1.1V,PCIEGEN1_TX_FS_3p5_DEEMPHASIS_1p2v
Model_198 3-STATE,1.1V,PCIEGEN1_TX_FS_3p5_DEEMPHASIS_0p8v
Model_199 3-STATE,1.1V,PCIEGEN1_TX_FS_3p5_DEEMPHASIS_0p6v
Model_200 3-STATE,1.1V,PCIEGEN1_TX_FS_3p5_DEEMPHASIS_0p4v
Model_201 3-STATE,1.1V,PCIEGEN1_TX_HS_NO_DEEMPHASIS_0p6v
Model_202 3-STATE,1.1V,PCIEGEN1_TX_HS_NO_DEEMPHASIS_0p4v
Model_203 3-STATE,1.1V,PCIEGEN1_TX_HS_NO_DEEMPHASIS_0p3v
Model_204 3-STATE,1.1V,PCIEGEN1_TX_HS_NO_DEEMPHASIS_0p2v
Model_205 3-STATE,1.1V,PCIEGEN2_TX_FS_NO_DEEMPHASIS_1p2v
Model_206 3-STATE,1.1V,PCIEGEN2_TX_FS_NO_DEEMPHASIS_0p8v
Model_207 3-STATE,1.1V,PCIEGEN2_TX_FS_NO_DEEMPHASIS_0p6v
Model_208 3-STATE,1.1V,PCIEGEN2_TX_FS_NO_DEEMPHASIS_0p4v
Model_209 3-STATE,1.1V,PCIEGEN2_TX_FS_3p5_DEEMPHASIS_1p2v
Model_210 3-STATE,1.1V,PCIEGEN2_TX_FS_3p5_DEEMPHASIS_0p8v
Model_211 3-STATE,1.1V,PCIEGEN2_TX_FS_3p5_DEEMPHASIS_0p6v
Model_212 3-STATE,1.1V,PCIEGEN2_TX_FS_3p5_DEEMPHASIS_0p4v
Model_213 3-STATE,1.1V,PCIEGEN2_TX_FS_6p0_DEEMPHASIS_1p2v
Model_214 3-STATE,1.1V,PCIEGEN2_TX_FS_6p0_DEEMPHASIS_0p8v
Model_215 3-STATE,1.1V,PCIEGEN2_TX_FS_6p0_DEEMPHASIS_0p6v
Model_216 3-STATE,1.1V,PCIEGEN2_TX_FS_6p0_DEEMPHASIS_0p4v
Model_217 3-STATE,1.1V,PCIEGEN2_TX_HS_NO_DEEMPHASIS_0p6v
Model_218 3-STATE,1.1V,PCIEGEN2_TX_HS_NO_DEEMPHASIS_0p4v
Model_219 3-STATE,1.1V,PCIEGEN2_TX_HS_NO_DEEMPHASIS_0p3v
Model_220 3-STATE,1.1V,PCIEGEN2_TX_HS_NO_DEEMPHASIS_0p2v
|   Usage I/O#1.8/3.3###BI2C1833DVFZP18_SSCEV.PAD
|   Base model BI2C1833DVFZP18_SSCEV
[Model Selector] Selector_3
Model_229 I/O_OPEN_DRAIN,1.8V,FAST MODE AND STD MODE,IND,10 PERCENT%,FAST_STD_MODE_1.8V_10P_1P8
Model_230 I/O_OPEN_DRAIN,3.3V,FAST MODE AND STD MODE,IND,10 PERCENT%,FAST_STD_MODE_3.3V_10P_3P3
Model_231 I/O_OPEN_DRAIN,1.8V,FAST MODE AND STD MODE,IND,5 PERCENT%,FAST_STD_MODE_1.8V_5P_1P8
Model_232 I/O_OPEN_DRAIN,3.3V,FAST MODE AND STD MODE,IND,5 PERCENT%,FAST_STD_MODE_3.3V_5P_3P3
|   Usage I/O#1.8/3.3###BC1833DV40DCPBFBP1811_SSCEH.PAD
|   Base model BC1833DV40DCPBFBP1811_SSCEH
[Model Selector] Selector_4
Model_168 I/O,1.8V,40D CLASS MODE FAST MODE,IND,10 PERCENT%,BC40D_H_10P_!SC1_1P8
Model_169 I/O,1.8V,40C CLASS MODE SLOW MODE,IND,10 PERCENT%,BC40D_H_10P_SC1_1P8
Model_170 I/O,1.8V,40D CLASS MODE FAST MODE,IND,5 PERCENT%,BC40D_H_5P_!SC1_1P8
Model_171 I/O,1.8V,40C CLASS MODE SLOW MODE,IND,5 PERCENT%,BC40D_H_5P_SC1_1P8
Model_172 I/O,3.3V,40D CLASS MODE FAST MODE,IND,10 PERCENT%,BC40D_H_10P_!SC1_3P3
Model_173 I/O,3.3V,40C CLASS MODE SLOW MODE,IND,10 PERCENT%,BC40D_H_10P_SC1_3P3
Model_174 I/O,3.3V,40D CLASS MODE FAST MODE,IND,5 PERCENT%,BC40D_H_5P_!SC1_3P3
Model_175 I/O,3.3V,40C CLASS MODE SLOW MODE,IND,5 PERCENT%,BC40D_H_5P_SC1_3P3
|   Usage I/O#1.35/1.5###DDR_DIFFIOPB_H.PADP
|   Base model DDR_DIFFIOPB_H
[Model Selector] Selector_5
Model_518 INPUT,1.5V,DDR3_ODT_80_1P5
Model_519 INPUT,1.5V,DDR3_ODT_60_1P5
Model_520 INPUT,1.5V,DDR3_ODT_120_1P5
Model_521 INPUT,1.35V,DDR3L_ODT_80_1P35
Model_522 INPUT,1.35V,DDR3L_ODT_60_1P35
Model_523 INPUT,1.35V,DDR3L_ODT_120_1P35
Model_527 I/O,1.5V,SR011_DRV40_1P5
Model_528 I/O,1.5V,SR010_DRV40_1P5
Model_529 I/O,1.5V,SR101_DRV40_1P5
Model_530 I/O,1.5V,SR100_DRV40_1P5
Model_531 I/O,1.5V,SR110_DRV40_1P5
Model_532 I/O,1.5V,SR111_DRV40_1P5
Model_533 I/O,1.5V,SR001_DRV40_1P5
Model_534 I/O,1.5V,SR000_DRV40_1P5
Model_535 I/O,1.5V,SR011_DRV34_1P5
Model_536 I/O,1.5V,SR010_DRV34_1P5
Model_537 I/O,1.5V,SR101_DRV34_1P5
Model_538 I/O,1.5V,SR100_DRV34_1P5
Model_539 I/O,1.5V,SR110_DRV34_1P5
Model_540 I/O,1.5V,SR111_DRV34_1P5
Model_541 I/O,1.5V,SR001_DRV34_1P5
Model_542 I/O,1.5V,SR000_DRV34_1P5
Model_543 I/O,1.5V,SR011_DRV48_1P5
Model_544 I/O,1.5V,SR010_DRV48_1P5
Model_545 I/O,1.5V,SR101_DRV48_1P5
Model_546 I/O,1.5V,SR100_DRV48_1P5
Model_547 I/O,1.5V,SR110_DRV48_1P5
Model_548 I/O,1.5V,SR111_DRV48_1P5
Model_549 I/O,1.5V,SR001_DRV48_1P5
Model_550 I/O,1.5V,SR000_DRV48_1P5
Model_551 I/O,1.35V,SR011_DRV40_1P35
Model_552 I/O,1.35V,SR010_DRV40_1P35
Model_553 I/O,1.35V,SR101_DRV40_1P35
Model_554 I/O,1.35V,SR100_DRV40_1P35
Model_555 I/O,1.35V,SR110_DRV40_1P35
Model_556 I/O,1.35V,SR111_DRV40_1P35
Model_557 I/O,1.35V,SR001_DRV40_1P35
Model_558 I/O,1.35V,SR000_DRV40_1P35
Model_559 I/O,1.35V,SR011_DRV34_1P35
Model_560 I/O,1.35V,SR010_DRV34_1P35
Model_561 I/O,1.35V,SR101_DRV34_1P35
Model_562 I/O,1.35V,SR100_DRV34_1P35
Model_563 I/O,1.35V,SR110_DRV34_1P35
Model_564 I/O,1.35V,SR111_DRV34_1P35
Model_565 I/O,1.35V,SR001_DRV34_1P35
Model_566 I/O,1.35V,SR000_DRV34_1P35
Model_567 I/O,1.35V,SR011_DRV48_1P35
Model_568 I/O,1.35V,SR010_DRV48_1P35
Model_569 I/O,1.35V,SR101_DRV48_1P35
Model_570 I/O,1.35V,SR100_DRV48_1P35
Model_571 I/O,1.35V,SR110_DRV48_1P35
Model_572 I/O,1.35V,SR111_DRV48_1P35
Model_573 I/O,1.35V,SR001_DRV48_1P35
Model_574 I/O,1.35V,SR000_DRV48_1P35
|   Usage OUTPUT#X###USB3_PCIEGEN1_PCIEGEN2_TX.TXP
|   Base model USB3_PCIEGEN1_PCIEGEN2_TX
[Model Selector] Selector_6
Model_190 3-STATE,1.1V,USB3_TX_FS_NO_DEEMPHASIS
Model_191 3-STATE,1.1V,USB3_TX_FS_3p5_DEEMPHASIS
Model_192 3-STATE,1.1V,USB3_TX_HS_NO_DEEMPHASIS
Model_193 3-STATE,1.1V,PCIEGEN1_TX_FS_NO_DEEMPHASIS_1p2v
Model_194 3-STATE,1.1V,PCIEGEN1_TX_FS_NO_DEEMPHASIS_0p8v
Model_195 3-STATE,1.1V,PCIEGEN1_TX_FS_NO_DEEMPHASIS_0p6v
Model_196 3-STATE,1.1V,PCIEGEN1_TX_FS_NO_DEEMPHASIS_0p4v
Model_197 3-STATE,1.1V,PCIEGEN1_TX_FS_3p5_DEEMPHASIS_1p2v
Model_198 3-STATE,1.1V,PCIEGEN1_TX_FS_3p5_DEEMPHASIS_0p8v
Model_199 3-STATE,1.1V,PCIEGEN1_TX_FS_3p5_DEEMPHASIS_0p6v
Model_200 3-STATE,1.1V,PCIEGEN1_TX_FS_3p5_DEEMPHASIS_0p4v
Model_201 3-STATE,1.1V,PCIEGEN1_TX_HS_NO_DEEMPHASIS_0p6v
Model_202 3-STATE,1.1V,PCIEGEN1_TX_HS_NO_DEEMPHASIS_0p4v
Model_203 3-STATE,1.1V,PCIEGEN1_TX_HS_NO_DEEMPHASIS_0p3v
Model_204 3-STATE,1.1V,PCIEGEN1_TX_HS_NO_DEEMPHASIS_0p2v
Model_205 3-STATE,1.1V,PCIEGEN2_TX_FS_NO_DEEMPHASIS_1p2v
Model_206 3-STATE,1.1V,PCIEGEN2_TX_FS_NO_DEEMPHASIS_0p8v
Model_207 3-STATE,1.1V,PCIEGEN2_TX_FS_NO_DEEMPHASIS_0p6v
Model_208 3-STATE,1.1V,PCIEGEN2_TX_FS_NO_DEEMPHASIS_0p4v
Model_209 3-STATE,1.1V,PCIEGEN2_TX_FS_3p5_DEEMPHASIS_1p2v
Model_210 3-STATE,1.1V,PCIEGEN2_TX_FS_3p5_DEEMPHASIS_0p8v
Model_211 3-STATE,1.1V,PCIEGEN2_TX_FS_3p5_DEEMPHASIS_0p6v
Model_212 3-STATE,1.1V,PCIEGEN2_TX_FS_3p5_DEEMPHASIS_0p4v
Model_213 3-STATE,1.1V,PCIEGEN2_TX_FS_6p0_DEEMPHASIS_1p2v
Model_214 3-STATE,1.1V,PCIEGEN2_TX_FS_6p0_DEEMPHASIS_0p8v
Model_215 3-STATE,1.1V,PCIEGEN2_TX_FS_6p0_DEEMPHASIS_0p6v
Model_216 3-STATE,1.1V,PCIEGEN2_TX_FS_6p0_DEEMPHASIS_0p4v
Model_217 3-STATE,1.1V,PCIEGEN2_TX_HS_NO_DEEMPHASIS_0p6v
Model_218 3-STATE,1.1V,PCIEGEN2_TX_HS_NO_DEEMPHASIS_0p4v
Model_219 3-STATE,1.1V,PCIEGEN2_TX_HS_NO_DEEMPHASIS_0p3v
Model_220 3-STATE,1.1V,PCIEGEN2_TX_HS_NO_DEEMPHASIS_0p2v
|   Usage I/O#1.8/3###SDIO1833PB_H.PAD
|   Base model SDIO1833PB_H
[Model Selector] Selector_7
Model_178 I/O,3V,50OHMS_3
Model_179 I/O,3V,66OHMS_3
Model_180 I/O,3V,33OHMS_3
Model_181 I/O,3V,100OHMS_3
Model_182 I/O,1.8V,50OHMS_1P8
Model_183 I/O,1.8V,66OHMS_1P8
Model_184 I/O,1.8V,33OHMS_1P8
Model_185 I/O,1.8V,100OHMS_1P8
|   Usage I/O#1.35/1.5###DDR_DIFFIOPB_H.PADN
|   Base model DDR_DIFFIOPB_H
[Model Selector] Selector_8
Model_518 INPUT,1.5V,DDR3_ODT_80_1P5
Model_519 INPUT,1.5V,DDR3_ODT_60_1P5
Model_520 INPUT,1.5V,DDR3_ODT_120_1P5
Model_521 INPUT,1.35V,DDR3L_ODT_80_1P35
Model_522 INPUT,1.35V,DDR3L_ODT_60_1P35
Model_523 INPUT,1.35V,DDR3L_ODT_120_1P35
Model_527 I/O,1.5V,SR011_DRV40_1P5
Model_528 I/O,1.5V,SR010_DRV40_1P5
Model_529 I/O,1.5V,SR101_DRV40_1P5
Model_530 I/O,1.5V,SR100_DRV40_1P5
Model_531 I/O,1.5V,SR110_DRV40_1P5
Model_532 I/O,1.5V,SR111_DRV40_1P5
Model_533 I/O,1.5V,SR001_DRV40_1P5
Model_534 I/O,1.5V,SR000_DRV40_1P5
Model_535 I/O,1.5V,SR011_DRV34_1P5
Model_536 I/O,1.5V,SR010_DRV34_1P5
Model_537 I/O,1.5V,SR101_DRV34_1P5
Model_538 I/O,1.5V,SR100_DRV34_1P5
Model_539 I/O,1.5V,SR110_DRV34_1P5
Model_540 I/O,1.5V,SR111_DRV34_1P5
Model_541 I/O,1.5V,SR001_DRV34_1P5
Model_542 I/O,1.5V,SR000_DRV34_1P5
Model_543 I/O,1.5V,SR011_DRV48_1P5
Model_544 I/O,1.5V,SR010_DRV48_1P5
Model_545 I/O,1.5V,SR101_DRV48_1P5
Model_546 I/O,1.5V,SR100_DRV48_1P5
Model_547 I/O,1.5V,SR110_DRV48_1P5
Model_548 I/O,1.5V,SR111_DRV48_1P5
Model_549 I/O,1.5V,SR001_DRV48_1P5
Model_550 I/O,1.5V,SR000_DRV48_1P5
Model_551 I/O,1.35V,SR011_DRV40_1P35
Model_552 I/O,1.35V,SR010_DRV40_1P35
Model_553 I/O,1.35V,SR101_DRV40_1P35
Model_554 I/O,1.35V,SR100_DRV40_1P35
Model_555 I/O,1.35V,SR110_DRV40_1P35
Model_556 I/O,1.35V,SR111_DRV40_1P35
Model_557 I/O,1.35V,SR001_DRV40_1P35
Model_558 I/O,1.35V,SR000_DRV40_1P35
Model_559 I/O,1.35V,SR011_DRV34_1P35
Model_560 I/O,1.35V,SR010_DRV34_1P35
Model_561 I/O,1.35V,SR101_DRV34_1P35
Model_562 I/O,1.35V,SR100_DRV34_1P35
Model_563 I/O,1.35V,SR110_DRV34_1P35
Model_564 I/O,1.35V,SR111_DRV34_1P35
Model_565 I/O,1.35V,SR001_DRV34_1P35
Model_566 I/O,1.35V,SR000_DRV34_1P35
Model_567 I/O,1.35V,SR011_DRV48_1P35
Model_568 I/O,1.35V,SR010_DRV48_1P35
Model_569 I/O,1.35V,SR101_DRV48_1P35
Model_570 I/O,1.35V,SR100_DRV48_1P35
Model_571 I/O,1.35V,SR110_DRV48_1P35
Model_572 I/O,1.35V,SR111_DRV48_1P35
Model_573 I/O,1.35V,SR001_DRV48_1P35
Model_574 I/O,1.35V,SR000_DRV48_1P35
|   Usage INPUT#1.8###CAMERARX_CORE.PADP
|   Base model CAMERARX_CORE
[Model Selector] Selector_9
Model_400 INPUT,1.8V,CAMERARX_CORE_HSRX
Model_401 INPUT,1.8V,CAMERARX_CORE_LPRX
Model_402 INPUT,1.8V,CAMERARX_CORE_ULPRX
Model_403 INPUT,1.8V,CAMERARX_CORE_PD_ON
Model_404 INPUT,1.8V,CAMERARX_CORE_PU_ON
Model_405 INPUT,1.8V,CAMERARX_CORE_PUPD0
|   Usage I/O#1.8/3.3###BC1833DV40DCPBFBP1811_SSCEV.PAD
|   Base model BC1833DV40DCPBFBP1811_SSCEV
[Model Selector] Selector_10
Model_752 I/O,1.8V,40D CLASS MODE FAST MODE,IND,10 PERCENT%,BC40D_V_10P_!SC1_1P8
Model_753 I/O,1.8V,40C CLASS MODE SLOW MODE,IND,10 PERCENT%,BC40D_V_10P_SC1_1P8
Model_754 I/O,1.8V,40D CLASS MODE FAST MODE,IND,5 PERCENT%,BC40D_V_5P_!SC1_1P8
Model_755 I/O,1.8V,40C CLASS MODE SLOW MODE,IND,5 PERCENT%,BC40D_V_5P_SC1_1P8
Model_756 I/O,3.3V,40D CLASS MODE FAST MODE,IND,10 PERCENT%,BC40D_V_10P_!SC1_3P3
Model_757 I/O,3.3V,40C CLASS MODE SLOW MODE,IND,10 PERCENT%,BC40D_V_10P_SC1_3P3
Model_758 I/O,3.3V,40D CLASS MODE FAST MODE,IND,5 PERCENT%,BC40D_V_5P_!SC1_3P3
Model_759 I/O,3.3V,40C CLASS MODE SLOW MODE,IND,5 PERCENT%,BC40D_V_5P_SC1_3P3
|   Usage OUTPUT#1.8/3.3###BC1833DV40DCPBFBHHVRXP1811_SSCEV.PAD
|   Base model BC1833DV40DCPBFBHHVRXP1811_SSCEV
[Model Selector] Selector_11
Model_762 I/O,1.8V,40D CLASS MODE FAST MODE,IND,10 PERCENT%,BC40DHHVRX_V_10P_!SC1_1P8
Model_763 I/O,1.8V,40C CLASS MODE SLOW MODE,IND,10 PERCENT%,BC40DHHVRX_V_10P_SC1_1P8
Model_764 I/O,1.8V,40D CLASS MODE FAST MODE,IND,5 PERCENT%,BC40DHHVRX_V_5P_!SC1_1P8
Model_765 I/O,1.8V,40C CLASS MODE SLOW MODE,IND,5 PERCENT%,BC40DHHVRX_V_5P_SC1_1P8
Model_766 I/O,3.3V,40D CLASS MODE FAST MODE,IND,10 PERCENT%,BC40DHHVRX_V_10P_!SC1_3P3
Model_767 I/O,3.3V,40C CLASS MODE SLOW MODE,IND,10 PERCENT%,BC40DHHVRX_V_10P_SC1_3P3
Model_768 I/O,3.3V,40D CLASS MODE FAST MODE,IND,5 PERCENT%,BC40DHHVRX_V_5P_!SC1_3P3
Model_769 I/O,3.3V,40C CLASS MODE SLOW MODE,IND,5 PERCENT%,BC40DHHVRX_V_5P_SC1_3P3
|   Usage INPUT#1.8/3.3###IHHV1833DVHYP1811_SSCEV.PAD
|   Base model IHHV1833DVHYP1811_SSCEV
[Model Selector] Selector_12
Model_233 INPUT,1.8V,1.8V MODE,IND,10 PERCENT%,IHHV1833_V_10P_1P8
Model_234 INPUT,3.3V,3.3V MODE,IND,10 PERCENT%,IHHV1833_V_10P_3P3
Model_235 INPUT,1.8V,1.8V MODE,IND,5 PERCENT%,IHHV1833_V_5P_1P8
Model_236 INPUT,3.3V,3.3V MODE,IND,5 PERCENT%,IHHV1833_V_5P_3P3
|   Usage OUTPUT#1.8/3.3###BC1833DV40DCPBFBP1811_SSCEV.PAD
|   Base model BC1833DV40DCPBFBP1811_SSCEV
[Model Selector] Selector_13
Model_752 I/O,1.8V,40D CLASS MODE FAST MODE,IND,10 PERCENT%,BC40D_V_10P_!SC1_1P8
Model_753 I/O,1.8V,40C CLASS MODE SLOW MODE,IND,10 PERCENT%,BC40D_V_10P_SC1_1P8
Model_754 I/O,1.8V,40D CLASS MODE FAST MODE,IND,5 PERCENT%,BC40D_V_5P_!SC1_1P8
Model_755 I/O,1.8V,40C CLASS MODE SLOW MODE,IND,5 PERCENT%,BC40D_V_5P_SC1_1P8
Model_756 I/O,3.3V,40D CLASS MODE FAST MODE,IND,10 PERCENT%,BC40D_V_10P_!SC1_3P3
Model_757 I/O,3.3V,40C CLASS MODE SLOW MODE,IND,10 PERCENT%,BC40D_V_10P_SC1_3P3
Model_758 I/O,3.3V,40D CLASS MODE FAST MODE,IND,5 PERCENT%,BC40D_V_5P_!SC1_3P3
Model_759 I/O,3.3V,40C CLASS MODE SLOW MODE,IND,5 PERCENT%,BC40D_V_5P_SC1_3P3
|   Usage INPUT#1.8###CAMERARX_CORE.PADN
|   Base model CAMERARX_CORE
[Model Selector] Selector_14
Model_400 INPUT,1.8V,CAMERARX_CORE_HSRX
Model_401 INPUT,1.8V,CAMERARX_CORE_LPRX
Model_402 INPUT,1.8V,CAMERARX_CORE_ULPRX
Model_403 INPUT,1.8V,CAMERARX_CORE_PD_ON
Model_404 INPUT,1.8V,CAMERARX_CORE_PU_ON
Model_405 INPUT,1.8V,CAMERARX_CORE_PUPD0
|   Usage INPUT#1.8/3.3###IQ1833DVTCKPBFBP18LL_SSCEV.PAD
|   Base model IQ1833DVTCKPBFBP18LL_SSCEV
[Model Selector] Selector_15
Model_186 INPUT,1.8V,1.8V MODE,IND,10 PERCENT%,IQ1833_V_10P_1P8
Model_187 INPUT,1.8V,1.8V MODE,IND,5 PERCENT%,IQ1833_V_5P_1P8
Model_188 INPUT,3.3V,3.3V MODE,IND,10 PERCENT%,IQ1833_V_10P_3P3
Model_189 INPUT,3.3V,3.3V MODE,IND,5 PERCENT%,IQ1833_V_5P_3P3
|   Usage INPUT#1.8###CAMERARX_ADDON.PADN
|   Base model CAMERARX_ADDON
[Model Selector] Selector_16
Model_408 INPUT,1.8V,CAMERARX_ADDON_HSRX
Model_409 INPUT,1.8V,CAMERARX_ADDON_LPRX
Model_410 INPUT,1.8V,CAMERARX_ADDON_ULPRX
Model_411 INPUT,1.8V,CAMERARX_ADDON_PD_ON
Model_412 INPUT,1.8V,CAMERARX_ADDON_PU_ON
Model_413 INPUT,1.8V,CAMERARX_ADDON_PUPD0
|   Usage INPUT#1.8###ILVDS18HY_SSCEH.PAD
|   Base model ILVDS18HY_SSCEH
[Model Selector] Selector_17
Model_5 INPUT,1.8V,LVDS MODE,IND,5%,LVDS_RX_MODE_5P_1P8
Model_6 INPUT,1.8V,LVDS MODE,IND,10%,LVDS_RX_MODE_10P_1P8
|   Usage INPUT#1.8/3.3###BC1833DV40DCPBFBP1811_SSCEV.PAD
|   Base model BC1833DV40DCPBFBP1811_SSCEV
[Model Selector] Selector_18
Model_752 I/O,1.8V,40D CLASS MODE FAST MODE,IND,10 PERCENT%,BC40D_V_10P_!SC1_1P8
Model_753 I/O,1.8V,40C CLASS MODE SLOW MODE,IND,10 PERCENT%,BC40D_V_10P_SC1_1P8
Model_754 I/O,1.8V,40D CLASS MODE FAST MODE,IND,5 PERCENT%,BC40D_V_5P_!SC1_1P8
Model_755 I/O,1.8V,40C CLASS MODE SLOW MODE,IND,5 PERCENT%,BC40D_V_5P_SC1_1P8
Model_756 I/O,3.3V,40D CLASS MODE FAST MODE,IND,10 PERCENT%,BC40D_V_10P_!SC1_3P3
Model_757 I/O,3.3V,40C CLASS MODE SLOW MODE,IND,10 PERCENT%,BC40D_V_10P_SC1_3P3
Model_758 I/O,3.3V,40D CLASS MODE FAST MODE,IND,5 PERCENT%,BC40D_V_5P_!SC1_3P3
Model_759 I/O,3.3V,40C CLASS MODE SLOW MODE,IND,5 PERCENT%,BC40D_V_5P_SC1_3P3
|   Usage OUTPUT#1.35/1.5###DDR_DIFFIOPB_V.PADN
|   Base model DDR_DIFFIOPB_V
[Model Selector] Selector_19
Model_690 I/O,1.5V,SR011_DRV40_1P5
Model_691 I/O,1.5V,SR010_DRV40_1P5
Model_692 I/O,1.5V,SR101_DRV40_1P5
Model_693 I/O,1.5V,SR100_DRV40_1P5
Model_694 I/O,1.5V,SR110_DRV40_1P5
Model_695 I/O,1.5V,SR111_DRV40_1P5
Model_696 I/O,1.5V,SR001_DRV40_1P5
Model_697 I/O,1.5V,SR000_DRV40_1P5
Model_698 I/O,1.5V,SR011_DRV34_1P5
Model_699 I/O,1.5V,SR010_DRV34_1P5
Model_700 I/O,1.5V,SR101_DRV34_1P5
Model_701 I/O,1.5V,SR100_DRV34_1P5
Model_702 I/O,1.5V,SR110_DRV34_1P5
Model_703 I/O,1.5V,SR111_DRV34_1P5
Model_704 I/O,1.5V,SR001_DRV34_1P5
Model_705 I/O,1.5V,SR000_DRV34_1P5
Model_706 I/O,1.5V,SR011_DRV48_1P5
Model_707 I/O,1.5V,SR010_DRV48_1P5
Model_708 I/O,1.5V,SR101_DRV48_1P5
Model_709 I/O,1.5V,SR100_DRV48_1P5
Model_710 I/O,1.5V,SR110_DRV48_1P5
Model_711 I/O,1.5V,SR111_DRV48_1P5
Model_712 I/O,1.5V,SR001_DRV48_1P5
Model_713 I/O,1.5V,SR000_DRV48_1P5
Model_714 I/O,1.35V,SR011_DRV40_1P35
Model_715 I/O,1.35V,SR010_DRV40_1P35
Model_716 I/O,1.35V,SR101_DRV40_1P35
Model_717 I/O,1.35V,SR100_DRV40_1P35
Model_718 I/O,1.35V,SR110_DRV40_1P35
Model_719 I/O,1.35V,SR111_DRV40_1P35
Model_720 I/O,1.35V,SR001_DRV40_1P35
Model_721 I/O,1.35V,SR000_DRV40_1P35
Model_722 I/O,1.35V,SR011_DRV34_1P35
Model_723 I/O,1.35V,SR010_DRV34_1P35
Model_724 I/O,1.35V,SR101_DRV34_1P35
Model_725 I/O,1.35V,SR100_DRV34_1P35
Model_726 I/O,1.35V,SR110_DRV34_1P35
Model_727 I/O,1.35V,SR111_DRV34_1P35
Model_728 I/O,1.35V,SR001_DRV34_1P35
Model_729 I/O,1.35V,SR000_DRV34_1P35
Model_730 I/O,1.35V,SR011_DRV48_1P35
Model_731 I/O,1.35V,SR010_DRV48_1P35
Model_732 I/O,1.35V,SR101_DRV48_1P35
Model_733 I/O,1.35V,SR100_DRV48_1P35
Model_734 I/O,1.35V,SR110_DRV48_1P35
Model_735 I/O,1.35V,SR111_DRV48_1P35
Model_736 I/O,1.35V,SR001_DRV48_1P35
Model_737 I/O,1.35V,SR000_DRV48_1P35
|   Usage I/O#X###USB2PHYCORE_HMAV10GS80.DP
|   Base model USB2PHYCORE_HMAV10GS80
[Model Selector] Selector_20
Model_738 3-STATE,3.3000V,fsdp_tx
Model_740 3-STATE,3.3000V,lsdp_50pf_tx
Model_742 3-STATE,3.3000V,lsdp_200pf_tx
Model_744 3-STATE,3.3000V,lsdp_400pf_tx
Model_746 3-STATE,3.3000V,lsdp_600pf_tx
Model_748 INPUT,3.3V,fsrx
Model_749 3-STATE,0.8000V,hsdp_tx
Model_751 INPUT,3.3V,hsrx
|   Usage INPUT#1.8###CAMERARX_ADDON.PADP
|   Base model CAMERARX_ADDON
[Model Selector] Selector_21
Model_408 INPUT,1.8V,CAMERARX_ADDON_HSRX
Model_409 INPUT,1.8V,CAMERARX_ADDON_LPRX
Model_410 INPUT,1.8V,CAMERARX_ADDON_ULPRX
Model_411 INPUT,1.8V,CAMERARX_ADDON_PD_ON
Model_412 INPUT,1.8V,CAMERARX_ADDON_PU_ON
Model_413 INPUT,1.8V,CAMERARX_ADDON_PUPD0
|   Usage OUTPUT#1.35/1.5###DDR_SEIOPB_V.PAD
|   Base model DDR_SEIOPB_V
[Model Selector] Selector_22
Model_350 I/O,1.5V,SR011_DRV40_1P5
Model_351 I/O,1.5V,SR010_DRV40_1P5
Model_352 I/O,1.5V,SR101_DRV40_1P5
Model_353 I/O,1.5V,SR100_DRV40_1P5
Model_354 I/O,1.5V,SR110_DRV40_1P5
Model_355 I/O,1.5V,SR111_DRV40_1P5
Model_356 I/O,1.5V,SR001_DRV40_1P5
Model_357 I/O,1.5V,SR000_DRV40_1P5
Model_358 I/O,1.5V,SR011_DRV34_1P5
Model_359 I/O,1.5V,SR010_DRV34_1P5
Model_360 I/O,1.5V,SR101_DRV34_1P5
Model_361 I/O,1.5V,SR100_DRV34_1P5
Model_362 I/O,1.5V,SR110_DRV34_1P5
Model_363 I/O,1.5V,SR111_DRV34_1P5
Model_364 I/O,1.5V,SR001_DRV34_1P5
Model_365 I/O,1.5V,SR000_DRV34_1P5
Model_366 I/O,1.5V,SR011_DRV48_1P5
Model_367 I/O,1.5V,SR010_DRV48_1P5
Model_368 I/O,1.5V,SR101_DRV48_1P5
Model_369 I/O,1.5V,SR100_DRV48_1P5
Model_370 I/O,1.5V,SR110_DRV48_1P5
Model_371 I/O,1.5V,SR111_DRV48_1P5
Model_372 I/O,1.5V,SR001_DRV48_1P5
Model_373 I/O,1.5V,SR000_DRV48_1P5
Model_374 I/O,1.35V,SR011_DRV40_1P35
Model_375 I/O,1.35V,SR010_DRV40_1P35
Model_376 I/O,1.35V,SR101_DRV40_1P35
Model_377 I/O,1.35V,SR100_DRV40_1P35
Model_378 I/O,1.35V,SR110_DRV40_1P35
Model_379 I/O,1.35V,SR111_DRV40_1P35
Model_380 I/O,1.35V,SR001_DRV40_1P35
Model_381 I/O,1.35V,SR000_DRV40_1P35
Model_382 I/O,1.35V,SR011_DRV34_1P35
Model_383 I/O,1.35V,SR010_DRV34_1P35
Model_384 I/O,1.35V,SR101_DRV34_1P35
Model_385 I/O,1.35V,SR100_DRV34_1P35
Model_386 I/O,1.35V,SR110_DRV34_1P35
Model_387 I/O,1.35V,SR111_DRV34_1P35
Model_388 I/O,1.35V,SR001_DRV34_1P35
Model_389 I/O,1.35V,SR000_DRV34_1P35
Model_390 I/O,1.35V,SR011_DRV48_1P35
Model_391 I/O,1.35V,SR010_DRV48_1P35
Model_392 I/O,1.35V,SR101_DRV48_1P35
Model_393 I/O,1.35V,SR100_DRV48_1P35
Model_394 I/O,1.35V,SR110_DRV48_1P35
Model_395 I/O,1.35V,SR111_DRV48_1P35
Model_396 I/O,1.35V,SR001_DRV48_1P35
Model_397 I/O,1.35V,SR000_DRV48_1P35
|   Usage OUTPUT#1.35/1.5###DDR_DIFFIOPB_V.PADP
|   Base model DDR_DIFFIOPB_V
[Model Selector] Selector_23
Model_690 I/O,1.5V,SR011_DRV40_1P5
Model_691 I/O,1.5V,SR010_DRV40_1P5
Model_692 I/O,1.5V,SR101_DRV40_1P5
Model_693 I/O,1.5V,SR100_DRV40_1P5
Model_694 I/O,1.5V,SR110_DRV40_1P5
Model_695 I/O,1.5V,SR111_DRV40_1P5
Model_696 I/O,1.5V,SR001_DRV40_1P5
Model_697 I/O,1.5V,SR000_DRV40_1P5
Model_698 I/O,1.5V,SR011_DRV34_1P5
Model_699 I/O,1.5V,SR010_DRV34_1P5
Model_700 I/O,1.5V,SR101_DRV34_1P5
Model_701 I/O,1.5V,SR100_DRV34_1P5
Model_702 I/O,1.5V,SR110_DRV34_1P5
Model_703 I/O,1.5V,SR111_DRV34_1P5
Model_704 I/O,1.5V,SR001_DRV34_1P5
Model_705 I/O,1.5V,SR000_DRV34_1P5
Model_706 I/O,1.5V,SR011_DRV48_1P5
Model_707 I/O,1.5V,SR010_DRV48_1P5
Model_708 I/O,1.5V,SR101_DRV48_1P5
Model_709 I/O,1.5V,SR100_DRV48_1P5
Model_710 I/O,1.5V,SR110_DRV48_1P5
Model_711 I/O,1.5V,SR111_DRV48_1P5
Model_712 I/O,1.5V,SR001_DRV48_1P5
Model_713 I/O,1.5V,SR000_DRV48_1P5
Model_714 I/O,1.35V,SR011_DRV40_1P35
Model_715 I/O,1.35V,SR010_DRV40_1P35
Model_716 I/O,1.35V,SR101_DRV40_1P35
Model_717 I/O,1.35V,SR100_DRV40_1P35
Model_718 I/O,1.35V,SR110_DRV40_1P35
Model_719 I/O,1.35V,SR111_DRV40_1P35
Model_720 I/O,1.35V,SR001_DRV40_1P35
Model_721 I/O,1.35V,SR000_DRV40_1P35
Model_722 I/O,1.35V,SR011_DRV34_1P35
Model_723 I/O,1.35V,SR010_DRV34_1P35
Model_724 I/O,1.35V,SR101_DRV34_1P35
Model_725 I/O,1.35V,SR100_DRV34_1P35
Model_726 I/O,1.35V,SR110_DRV34_1P35
Model_727 I/O,1.35V,SR111_DRV34_1P35
Model_728 I/O,1.35V,SR001_DRV34_1P35
Model_729 I/O,1.35V,SR000_DRV34_1P35
Model_730 I/O,1.35V,SR011_DRV48_1P35
Model_731 I/O,1.35V,SR010_DRV48_1P35
Model_732 I/O,1.35V,SR101_DRV48_1P35
Model_733 I/O,1.35V,SR100_DRV48_1P35
Model_734 I/O,1.35V,SR110_DRV48_1P35
Model_735 I/O,1.35V,SR111_DRV48_1P35
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| Models and submodels in the file (323): Model_1 (Input), Model_2 (Input), Model_3 (3-state), Model_4 (3-state), Model_5 (Input), Model_6 (Input), Model_111 (Input), Model_112 (Input), Model_113 (Input), Model_114 (Input), Model_115 (Input), Model_116 (Input), Model_120 (I/O), Model_121 (I/O), Model_122 (I/O), Model_123 (I/O), Model_124 (I/O), Model_125 (I/O), Model_126 (I/O), Model_127 (I/O), Model_128 (I/O), Model_129 (I/O), Model_130 (I/O), Model_131 (I/O), Model_132 (I/O), Model_133 (I/O), Model_134 (I/O), Model_135 (I/O), Model_136 (I/O), Model_137 (I/O), Model_138 (I/O), Model_139 (I/O), Model_140 (I/O), Model_141 (I/O), Model_142 (I/O), Model_143 (I/O), Model_144 (I/O), Model_145 (I/O), Model_146 (I/O), Model_147 (I/O), Model_148 (I/O), Model_149 (I/O), Model_150 (I/O), Model_151 (I/O), Model_152 (I/O), Model_153 (I/O), Model_154 (I/O), Model_155 (I/O), Model_156 (I/O), Model_157 (I/O), Model_158 (I/O), Model_159 (I/O), Model_160 (I/O), Model_161 (I/O), Model_162 (I/O), Model_163 (I/O), Model_164 (I/O), Model_165 (I/O), Model_166 (I/O), Model_167 (I/O), Model_168 (I/O), Model_169 (I/O), Model_170 (I/O), Model_171 (I/O), Model_172 (I/O), Model_173 (I/O), Model_174 (I/O), Model_175 (I/O), Model_177 (Input), Model_178 (I/O), Model_179 (I/O), Model_180 (I/O), Model_181 (I/O), Model_182 (I/O), Model_183 (I/O), Model_184 (I/O), Model_185 (I/O), Model_186 (Input), Model_187 (Input), Model_188 (Input)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
